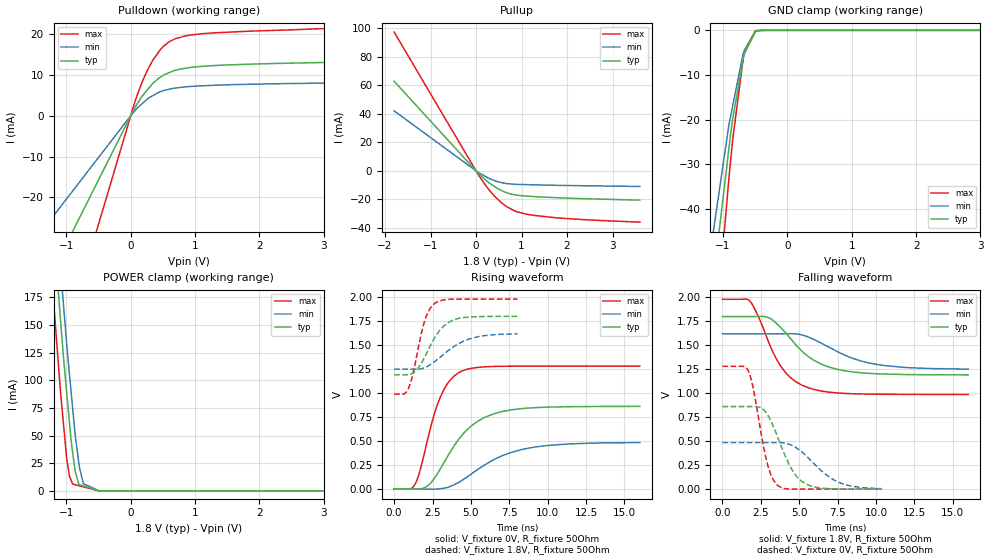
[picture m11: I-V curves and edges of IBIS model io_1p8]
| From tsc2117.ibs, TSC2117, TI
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|   io_1p8 Model
[Model]   io_1p8
Model_type   I/O
Polarity   Non-Inverting
Enable   Active-High
Vinl = 0.54
Vinh = 1.26
Vmeas = 0.9
Vref = 0.9
Cref = 10pF
Rref = 50
|   typ   min   max
|   (nom PVT)   (fast PVT)   (slow PVT)
|C_comp from frequency sweep method (F=14MHz)
|Average
|C_comp   3.364e-12   3.163e-12   3.372e-12
|ON state : BUFFER OUTPUT TURNED HIGH
|C_comp   4.691e-12   4.325e-12   4.717e-12
|OFF state: BUFFER IN HIGH IMPEDANCE
|C_comp   2.028e-12   2.001e-12   2.036e-12
|C_comp from LC tank measurement(L=1nH)
|Average
|Resonant Frequency(Hz)   4.160e+09   4.200e+09   4.125e+09
C_comp   1.467e-12   1.439e-12   1.494e-12
|ON state : BUFFER OUTPUT TURNED HIGH
|Resonant Frequency(Hz)   4.070e+09   4.130e+09   4.010e+09
|C_comp   1.531e-12   1.487e-12   1.577e-12
|OFF state: BUFFER IN HIGH IMPEDANCE
|Resonant Frequency(Hz)   4.250e+09   4.270e+09   4.240e+09
|C_comp   1.404e-12   1.391e-12   1.410e-12
| Where nom  PVT is Nominal Process, 1.8V, 48C
|   Fast PVT is Strong Process,  1.98V, -40C
|   Slow PVT is Weak Process,   1.62V, 108C
[Model Spec]
|Subparameter   typ   min   max
Vinh   1.26   1.134   1.386
Vinl   0.54   0.486   0.594
[Voltage Range]   1.8   1.62   1.98
|Ambient Temperature   25   85   -40
|Junction Temperature
[Temperature Range]   48   108   -40
[Pullup Reference]   1.8   1.62   1.98
[Pulldown Reference]   0   0   0
[Power Clamp Reference]   1.8   1.62   1.98
[GND Clamp Reference]   0   0   0
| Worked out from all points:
|   slope of the pulldown table from 0 to 0.27 V, typ, clamps not added: 41.3 ohm
|   slope of the pullup table from 0 to 0.27 V, typ, clamps not added: 34 ohm
|   GND clamp passes 1 mA (typ) near -0.52 V on its own axis
|   POWER clamp passes 1 mA (typ) near -0.54 V on its own axis
|   falling waveform, V_fixture 1.8V, R_fixture 50Ohm: 20-80 % time 2.48ns typ, 3.16ns min, 1.9ns max; typ from 1.8 V to 1.19 V
|   rising waveform, V_fixture 0V, R_fixture 50Ohm: 20-80 % time 2.42ns typ, 3.28ns min, 1.42ns max; typ from 0 V to 0.861 V
|   rising waveform, V_fixture 1.8V, R_fixture 50Ohm: 20-80 % time 1.34ns typ, 1.98ns min, 845ps max; typ from 1.19 V to 1.8 V
|   falling waveform, V_fixture 0V, R_fixture 50Ohm: 20-80 % time 1.43ns typ, 2.05ns min, 903ps max; typ from 0.861 V to 0 V
[Pulldown]
|   Voltage   I(typ)   I(min)   I(max)
-1.8V     -56.49mA   -36.75mA   -95.55mA
-72mV     -2.259mA   -1.47mA    -3.822mA
95.04mV   2.758mA    1.751mA    4.798mA
168.3mV   4.552mA    2.822mA    7.911mA
251.5mV   6.192mA    3.988mA    10.89mA
348.5mV   7.968mA    4.952mA    13.71mA
463.3mV   9.448mA    5.897mA    16.21mA
601.9mV   10.55mA    6.481mA    18.13mA
698.9mV   11.15mA    6.779mA    18.88mA
855.4mV   11.62mA    7.059mA    19.53mA
1.277V    12.25mA    7.427mA    20.26mA
3.6V      13.28mA    8.129mA    21.69mA
[GND Clamp]
|   Voltage   I(typ)   I(min)   I(max)
-1.8V     -204.6mA   -123mA     -346.6mA
-1.166V   -57.91mA   -46.59mA   -76.42mA
-910.4mV  -26.62mA   -21.3mA    -33.38mA
-883.8mV  -23.36mA   -19.36mA   -29.42mA
-849.4mV  -19.83mA   -16.88mA   -24.37mA
-686.9mV  -6.332mA   -5.148mA   -6.348mA
-676.8mV  -5.495mA   -4.894mA   -5.23mA
-671.2mV  -5.334mA   -4.752mA   -4.611mA
-495mV    -237.7uA   -296.5uA   -66.69uA
-307.8mV  -1.3uA     -3.437uA   -91.66nA
3.6V      0A         0A         0A
[Pullup]
|   Voltage   I(typ)   I(min)   I(max)
-1.8V     62.74mA    41.98mA    97.18mA
95.04mV   -3.093mA   -1.942mA   -4.857mA
348.5mV   -9.775mA   -6.119mA   -15.69mA
601.9mV   -14.42mA   -8.513mA   -23.45mA
683.1mV   -15.42mA   -8.991mA   -25.3mA
900.9mV   -17.04mA   -9.476mA   -28.73mA
1.277V    -18.04mA   -9.812mA   -31.23mA
2.376V    -19.52mA   -10.46mA   -34.22mA
3.6V      -20.5mA    -10.94mA   -35.98mA
[POWER Clamp]
|   Voltage   I(typ)   I(min)   I(max)
-1.8V     711.3mA    747.3mA    662mA
-1.215V   245.7mA    292.3mA    183mA
-1.129V   182.6mA    228.3mA    118.2mA
-1.044V   120mA      167.5mA    59.76mA
-994mV    88.16mA    131.9mA    28.81mA
-952.4mV  61.74mA    105.3mA    13.13mA
-902.9mV  34.89mA    74.83mA    6.212mA
-865.8mV  18.41mA    52.09mA    5.654mA
-806.4mV  5.838mA    25.14mA    4.761mA
-737.1mV  4.574mA    6.658mA    3.718mA
-494.1mV  154.3uA    103.9uA    74.57uA
3.6V      0A         0A         0A
[Ramp]
R_load = 50
|   typ   min   max
dV/dt_r   0.516391/2.41299e-09   0.290194/3.26051e-09   0.768593/1.41272e-09
dV/dt_f   0.364978/2.47197e-09   0.22121/3.15648e-09   0.595433/1.89507e-09
[Falling Waveform]
V_fixture = 1.8V
V_fixture_min = 1.62V
V_fixture_max = 1.98V
R_fixture = 50Ohm
|   Time   V(typ)   V(min)   V(max)
0s        1.8V       1.62V      1.98V
1.776ns   1.8V       1.62V      1.963V
2.204ns   1.8V       1.62V      1.846V
2.829ns   1.798V     1.62V      1.606V
3.768ns   1.689V     1.62V      1.289V
4.52ns    1.554V     1.621V     1.151V
5.445ns   1.401V     1.595V     1.066V
7.25ns    1.258V     1.454V     1.006V
9.629ns   1.206V     1.313V     990.5mV
16ns      1.192V     1.251V     987.6mV
[Rising Waveform]
V_fixture = 0V
V_fixture_min = 0V
V_fixture_max = 0V
R_fixture = 50Ohm
|   Time   V(typ)   V(min)   V(max)
0s        2.105nV    9.045nV    579.6pV
1.362ns   -2.144mV   63.93uV    48.57mV
1.659ns   -844.8uV   -279.9uV   176.8mV
2.184ns   32.71mV    -1.569mV   518.5mV
2.956ns   195.2mV    1.035mV    936.6mV
3.576ns   365.6mV    21.68mV    1.121V
4.319ns   540.8mV    79.59mV    1.222V
5.892ns   745.5mV    250.2mV    1.273V
8.316ns   837.8mV    411.2mV    1.28V
16ns      860.7mV    483.7mV    1.281V
[Rising Waveform]
V_fixture = 1.8V
V_fixture_min = 1.62V
V_fixture_max = 1.98V
R_fixture = 50Ohm
|   Time   V(typ)   V(min)   V(max)
0s        1.191V     1.249V     987.6mV
641ps     1.191V     1.249V     989.2mV
914ps     1.191V     1.249V     1.043V
1.209ns   1.206V     1.249V     1.189V
1.975ns   1.371V     1.264V     1.745V
2.651ns   1.58V      1.329V     1.935V
3.314ns   1.71V      1.416V     1.974V
4.186ns   1.778V     1.514V     1.98V
5.83ns    1.798V     1.598V     1.98V
8.043ns   1.8V       1.618V     1.98V
[Falling Waveform]
V_fixture = 0V
V_fixture_min = 0V
V_fixture_max = 0V
R_fixture = 50Ohm
|   Time   V(typ)   V(min)   V(max)
0s        860.8mV    485.3mV    1.281V
1.686ns   860.8mV    485.3mV    1.233V
2.011ns   860.9mV    485.3mV    1.045V
2.876ns   790.3mV    485.3mV    293.8mV
3.233ns   683.8mV    485.3mV    120.9mV
3.571ns   552.4mV    485.4mV    41.98mV
4.52ns    204.4mV    456.4mV    -860.2uV
5.408ns   55.79mV    353mV      642uV
7.678ns   1.57mV     63.41mV    192.8uV
10.38ns   199uV      3.987mV    34.31uV
